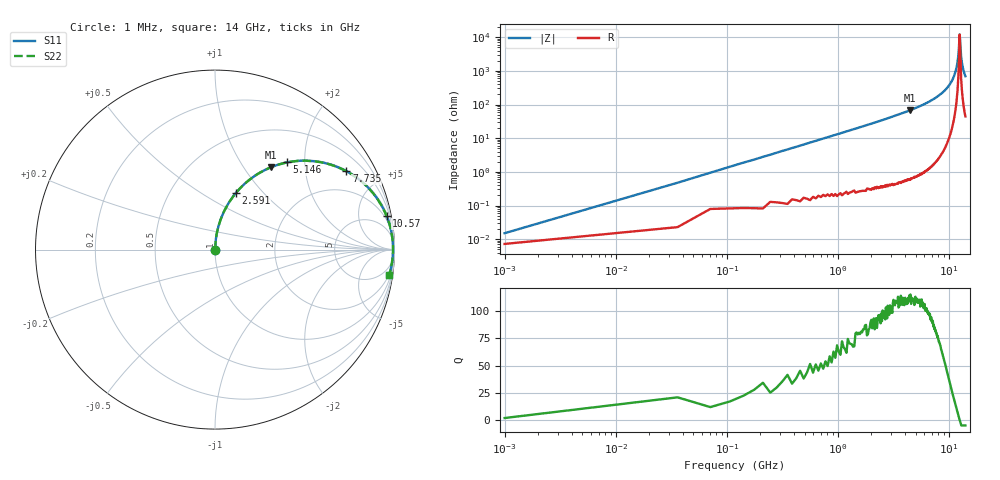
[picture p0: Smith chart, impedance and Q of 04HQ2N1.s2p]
! Coilcraft 0403HQ-2N1 Chip Inductor
! 13 February 2004
# MHZ S MA R 50
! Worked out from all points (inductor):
!   401 points, 1 MHz to 14 GHz, reference 50 ohm
!   read as one part in series: L = 2.1 nH near 71 MHz
!   highest Q = 112 at 4.446 GHz (marker M1), where L = 2.41 nH
!   self-resonance near 12.43 GHz
!   S11 on the Smith chart (normalised r, x): 1 MHz: 1.00, +0.00; 2.591 GHz: 1.01, +0.71; 5.146 GHz: 1.01, +1.64; 7.735 GHz: 1.05, +3.33; 10.57 GHz: 1, +10; 14 GHz: 2, -14
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1  0.0001957 42.4  1 -0.0  1 -0.0  0.0001957 42.4
105.992  0.014 86.2  0.999 -0.8  0.999 -0.8  0.014 86.2
210.985  0.028 86.3  0.999 -1.6  0.999 -1.6  0.028 86.3
385.972  0.051 85.6  0.997 -2.9  0.997 -2.9  0.051 85.6
1085.922  0.143 80.9  0.988 -8.2  0.988 -8.2  0.143 80.9
2345.832  0.305 71.6  0.949 -17.7  0.949 -17.7  0.305 71.6
2590.815  0.335 69.8  0.939 -19.6  0.939 -19.6  0.335 69.8
4445.682  0.556 55.7  0.826 -33.8  0.826 -33.8  0.556 55.7
4690.665  0.583 53.8  0.807 -35.6  0.807 -35.6  0.583 53.8
5145.633  0.631 50.4  0.77 -39.1  0.77 -39.1  0.631 50.4
7000.5  0.8 36.3  0.591 -53.1  0.591 -53.1  0.8 36.3
7735.448  0.852 30.8  0.512 -58.5  0.512 -58.5  0.852 30.8
9345.333  0.937 19.3  0.331 -69.5  0.331 -69.5  0.937 19.3
10570.25  0.974 11.2  0.194 -76.7  0.194 -76.7  0.974 11.2
11690.17  0.989 4.3  0.075 -79.8  0.075 -79.8  0.989 4.3
12075.14  0.991 2.0  0.036 -75.3  0.036 -75.3  0.991 2.0
12425.11  0.992 0.1  0.008241 -7.3  0.008241 -7.3  0.992 0.1
12495.11  0.992 -0.3  0.01 34.6  0.01 34.6  0.992 -0.3
12740.09  0.991 -1.7  0.03 72.4  0.03 72.4  0.991 -1.7
12985.07  0.99 -3.0  0.053 77.8  0.053 77.8  0.99 -3.0
13405.04  0.987 -5.2  0.091 79.3  0.091 79.3  0.987 -5.2
14000  0.981 -8.2  0.142 78.2  0.142 78.2  0.981 -8.2
